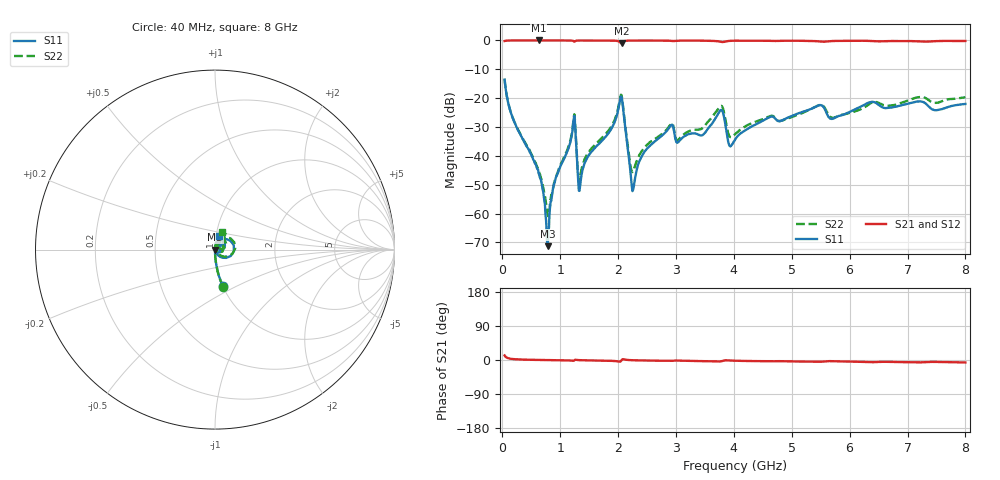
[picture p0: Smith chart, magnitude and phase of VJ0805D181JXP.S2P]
! VJ0805D181JXP
! DATE 03/14/2022  09:01
! CAPACITORS MOUNTED IN SERIES ON 25 MIL THICK MICROSTRIP SUBSTRATE
# GHz  S  MA  R  50.00
!  FREQ  S11M  S11A  S21M  S21A  S12M  S12A  S22M  S22A
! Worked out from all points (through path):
!   801 points, 40 MHz to 8 GHz, reference 50 ohm
!   highest |S21| = 0.00 dB at 627 MHz (marker M1); lowest = -1.0 dB at 2.06 GHz (marker M2)
!   group delay of S21, straight-line fit = 2.55 ps
!   lowest |S11| = -71.3 dB at 786.2 MHz (marker M3), VSWR 1.00, Z = 50 - j0.00179 ohm
!   |S11| at or under -10 dB: start of sweep to end of sweep
!   |S22| runs from -61.0 to -13.4 dB; largest |S21 - S12| = 0.0032
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0.04  0.21 -77.7  0.9778 12.1  0.9765 12.1  0.2128 -78.0
0.18925  0.0428 -87.6  0.9989 2.4  0.9986 2.5  0.04338 -87.5
0.62705  0.005084 -87.5  0.9999 0.2  0.9999 0.1  0.005588 -83.0
0.78625  0.0002728 -3.8  0.9994 -0.2  0.9996 -0.2  0.0009428 -13.7
0.90565  0.003494 84.4  0.9994 -0.4  0.9996 -0.4  0.003706 68.9
1.22405  0.03476 58.9  0.9824 -2.1  0.9826 -2.1  0.03717 58.7
1.32355  0.002483 1.9  0.9971 -0.3  0.9973 -0.3  0.003749 10.9
1.3733  0.00497 72.6  0.9984 -0.6  0.9986 -0.6  0.006177 65.3
2.05985  0.1058 -5.4  0.8916 -0.5  0.892 -0.5  0.1127 3.1
2.25885  0.002583 14.2  0.9965 -0.6  0.9972 -0.7  0.005375 26.3
2.41805  0.01024 75.3  0.9979 -1.2  0.998 -1.2  0.01245 73.4
2.69665  0.02003 75.4  0.9966 -1.9  0.9972 -1.9  0.02171 77.7
2.91555  0.03413 54.8  0.9848 -2.5  0.9845 -2.5  0.03611 62.1
3.03495  0.01719 51.1  0.9929 -1.6  0.9939 -1.7  0.01877 60.2
3.45285  0.02273 66.7  0.9919 -3.1  0.9922 -3.1  0.03003 79.1
3.77125  0.06189 42.5  0.9495 -3.6  0.9496 -3.6  0.07323 47.2
3.93045  0.0148 28.0  0.9832 -1.3  0.984 -1.3  0.02143 31.3
4.02995  0.01973 64.0  0.9906 -1.9  0.9905 -2.0  0.0243 61.4
5.3533  0.0663 63.3  0.9782 -4.6  0.9784 -4.7  0.06648 70.0
5.6916  0.04364 51.6  0.9759 -3.1  0.9759 -3.1  0.04597 50.9
6.67665  0.06801 67.4  0.9752 -4.9  0.9754 -5.0  0.07414 60.0
8  0.07933 74.2  0.9793 -6.5  0.979 -6.5  0.1039 67.9
